FUNCTION_BLOCK PQDXXA_PFN
TITLE =PN Driver
AUTHOR : Parker
VERSION : 1.1


VAR_INPUT
  ENABLE : BOOL ;	//Freigabe des Systems / Enable the System
  ENABLE_P : BOOL ;	//Aktivierung des Druckreglers / Activation of the Pressure Controller
  ENABLE_RAMP : BOOL ;	//Aktivierung des Rampengenerators / Activation of the Ramp Generator
  ENABLE_PL : BOOL ;	//Freigabe der Leistungsbegrenzung über den Feldbus / Enable the Power Limitation
  WQ : REAL ;	//Schwenkwinkelsollwert [%] / Displacement Command Value [%]
  WP : REAL  := 1.000000e+002;	//Drucksollwert [bar] / Pressure Command Value [bar]
  WL : REAL ;	//Leistungssollwert [%] / Horse Power Command [%]
  PAR_CHANGE_IN : STRUCT
   PARVAL : DWORD ;
   PARAMODE : BOOL ;
   ADDRESS : WORD ;
   PARAVALID : BOOL ;
   PARAREAD : BOOL ;
   READULIM : BOOL ;
   READLLIM : BOOL ;
  END_STRUCT ;
  ADR_IN : INT ;	//Eingangsadresse des Slaves / Input adress of the slave
  ADR_OUT : INT ;	//Ausgangsadresse des Slaves / Output adress of the slave
END_VAR
VAR_OUTPUT
  BUS_VALID : BOOL ;	//Buskopplung liefert gültige Werte / Bus Connection Delivers Valid Information
  BUS_ERROR_CODE : BYTE ;	//Fehlercode zur Diagnose / Error Code for Diagnosis
  ERROR : BOOL ;	//Sammelfehler / Common Error Bit
  P_ACTIVE : BOOL ;	//Druckregler aktiv / Pressure Controller Active
  POWER_LIM : BOOL ;	//Leistungsbegrenzung Aktiv / Horse Power Limitation is Active
  READY : BOOL ;	//Allgemeine Betriebsbereitschaft / Operational Readiness
  IQA_ERROR : BOOL ;	//Fehler Magnet A / Error Solenoid A
  IQB_ERROR : BOOL ;	//Fehler Magnet B / Error Solenoid B
  IP_ERROR : BOOL ;	//Fehler Druckventil / Error Pressure Valve
  XQ_ERROR : BOOL ;	//Fehler Schwenkwinkelsensor / Error Displacement Transducer
  XP_ERROR : BOOL ;	//Fehler Drucksensor / Error Pressure Transducer
  HW_ENABLE : BOOL ;	//Enable Eingang des Moduls an PIN8 / Enable Input of the Module at PIN8
  WQFB : REAL ;	//Schwenkwinkelsollwert [%] Rückmeldung / Displacement Command Value [%] Feedback
  XQ : REAL ;	//Schwenkwinkelistwert [%] / Displacement Actual Value [%]
  EQ : REAL ;	//Regelabweichung Schwenkwinkel [%] / Control Error Displacement [%]
  UQ : REAL ;	//Stellsignal Q Ventil [%] / Control Signal Q Valve [%]
  WPFB : REAL ;	//Drucksollwert [bar] Rückmeldung / Pressure Command Value [%] Feedback
  XP : REAL ;	//Druckistwert [bar] / Pressure Actual Value [bar]
  EP : REAL ;	//Regelabweichung Druck [bar] / Control Error Pressure [bar]
  UP : REAL ;	//Stellsignal P Ventil [%] / Control Signal P Valve [%]
  XL : REAL ;	//Schwenkwinkelgrenze durch Leistung [%] / Displacement Limit by Power [%]
  XQ_R : REAL ;	//Schwenkwinkelsensorsignal [V] / Displacement Sensor Signal [V]
  IQ : REAL ;	//Magnetstrom Schwenkwinkelventil [mA] / Solenoid Current Displacement Valve [mA]
  IP : REAL ;	//Magnetstrom Druckventil [mA] / Solenoid Current Pressure Valve [mA]
  PAR_CHANGE_OUT : STRUCT
   PARA_READY : BOOL ;
   BUS_VALID : BOOL ;
   ENABLE : BOOL ;	//Enable Signal for the Controller
   PARA_ACTIVE : BOOL ;
   PARVAL : DWORD ;	//Read out Value
  END_STRUCT ;
END_VAR
VAR
  DATA_IN : ARRAY  [0 .. 31 ] OF BYTE ;
  DATA_OUT : ARRAY  [0 .. 31 ] OF BYTE ;
  LIVEBIT : BOOL ;
  ERROR_TIMER_ON : INT ;
  ERROR_TIMER_OFF : INT ;
END_VAR
VAR_TEMP
  RET_VAL_TMP : INT ;
  TMP_VAL : DWORD ;
  TMP_VAL_WORD : WORD ;
  TMP_BYTE : BYTE ;
  TMP_VAL_REAL : REAL ;
  RCV_ERROR : BOOL ;
  SND_ERROR : BOOL ;
  LIVEBIT_ERROR : BOOL ;
  BUFFERR0V : BOOL ;
  CHKERROR : BOOL ;
  DERROR : BOOL ;
  LIVEBIT_FB : BOOL ;
  i : INT ;
  ADRE : WORD ;
END_VAR
BEGIN
NETWORK
TITLE =

      SET   ;
      SAVE  ;
      =     L     20.1;
      L     #ADR_IN;
      T     #ADRE;
      SAVE  ;

      CALL SFC   14 (
           LADDR                    := #ADRE,
           RET_VAL                  := #RET_VAL_TMP,
           RECORD                   := #DATA_IN);

      L     #RET_VAL_TMP;
      L     0;
      <>I   ;
      =     #RCV_ERROR;
      L     #DATA_IN[0];
      T     #TMP_BYTE;
      U     L      8.0;
      NOT   ;
      =     #DERROR;
      U     L      8.1;
      NOT   ;
      =     #CHKERROR;
      U     L      8.2;
      NOT   ;
      =     #BUFFERR0V;
      U     L      8.3;
      =     #HW_ENABLE;
      U     L      8.4;
      NOT   ;
      =     #ERROR;
      U     L      8.5;
      =     #P_ACTIVE;
      U     L      8.6;
      =     #POWER_LIM;
      U     L      8.7;
      =     #READY;
      U     #ENABLE;
      =     #PAR_CHANGE_OUT.ENABLE;
      L     #DATA_IN[1];
      T     #TMP_BYTE;
      U     L      8.0;
      =     #LIVEBIT_FB;
      U     L      8.1;
      NOT   ;
      =     #IQA_ERROR;
      U     L      8.2;
      NOT   ;
      =     #IQB_ERROR;
      U     L      8.3;
      NOT   ;
      =     #IP_ERROR;
      U     L      8.4;
      NOT   ;
      =     #XQ_ERROR;
      U     L      8.5;
      NOT   ;
      =     #XP_ERROR;
      U     L      8.6;
      =     #PAR_CHANGE_OUT.PARA_READY;
      U     L      8.7;
      =     #PAR_CHANGE_OUT.PARA_ACTIVE;
      U     #LIVEBIT;
      X     #LIVEBIT_FB;
      SPBN  A7d0;
      L     #ERROR_TIMER_ON;
      L     1;
      +I    ;
      SPO   I007;
      SPA   I008;
I007: CLR   ;
      =     L     20.1;
I008: T     #ERROR_TIMER_ON;
      SPA   A7d1;
A7d0: CLR   ;
      U     #LIVEBIT;
      NOT   ;
      =     #LIVEBIT;
      L     0;
      T     #ERROR_TIMER_ON;
A7d1: L     #ERROR_TIMER_ON;
      L     10;
      >=I   ;
      SPBN  A7d2;
      U     #LIVEBIT;
      NOT   ;
      =     #LIVEBIT;
      L     0;
      T     #ERROR_TIMER_ON;
      L     25;
      T     #ERROR_TIMER_OFF;
A7d2: L     #ERROR_TIMER_OFF;
      L     0;
      >I    ;
      SPBN  A7d3;
      L     #ERROR_TIMER_OFF;
      L     1;
      -I    ;
      SPO   I009;
      SPA   I00a;
I009: CLR   ;
      =     L     20.1;
I00a: T     #ERROR_TIMER_OFF;
      SET   ;
      =     #LIVEBIT_ERROR;
      SPA   A7d4;
A7d3: CLR   ;
      =     #LIVEBIT_ERROR;
A7d4: L     0;
      T     #i;
A7d5: L     #i;
      L     1;
      <=I   ;
      SPBN  A7d6;
      L     #i;
      +I    ;
      SPO   I00b;
      SPA   I00c;
I00b: CLR   ;
      =     L     20.1;
I00c: ITD   ;
      L     L#1;
      >=D   ;
      U     L     20.1;
      =     L     20.1;
      TAK   ;
      L     L#2;
      <=D   ;
      U     L     20.1;
      =     L     20.1;
      TAK   ;
      L     L#1;
      -D    ;
      SPO   I00d;
      SPA   I00e;
I00d: CLR   ;
      =     L     20.1;
I00e: L     L#8;
      *D    ;
      SPO   I00f;
      SPA   I010;
I00f: CLR   ;
      =     L     20.1;
I010: L     4;
      TAK   ;
      T     LD    22;
      TAK   ;
      L     #i;
      +I    ;
      SPO   I011;
      SPA   I012;
I011: CLR   ;
      =     L     20.1;
I012: ITD   ;
      L     L#0;
      >=D   ;
      U     L     20.1;
      =     L     20.1;
      TAK   ;
      L     L#31;
      <=D   ;
      U     L     20.1;
      =     L     20.1;
      TAK   ;
      L     L#8;
      *D    ;
      SPO   I013;
      SPA   I014;
I013: CLR   ;
      =     L     20.1;
I014: TAR2  ;
      +D    ;
      SPO   I015;
      SPA   I016;
I015: CLR   ;
      =     L     20.1;
I016: LAR1  ;
      L     DIB [AR1,P#86.0];
      LAR1  LD    22;
      T     LB [AR1,P#6.0];
      L     #i;
      L     1;
      +I    ;
      SPO   I017;
      SPA   I018;
I017: CLR   ;
      =     L     20.1;
I018: T     #i;
      SPA   A7d5;
A7d6: L     #TMP_VAL_WORD;
      CLR   ;
      U     L     20.1;
      SAVE  ;
      ITD   ;
      DTR   ;
      T     #TMP_VAL_REAL;
      SAVE  ;
      L     1.638300e+002;
      /R    ;
      SPO   I019;
      SPA   I01a;
I019: CLR   ;
      =     L     20.1;
I01a: T     #WQFB;
      L     0;
      T     #i;
A7d7: L     #i;
      L     1;
      <=I   ;
      SPBN  A7d8;
      L     #i;
      +I    ;
      SPO   I01b;
      SPA   I01c;
I01b: CLR   ;
      =     L     20.1;
I01c: ITD   ;
      L     L#1;
      >=D   ;
      U     L     20.1;
      =     L     20.1;
      TAK   ;
      L     L#2;
      <=D   ;
      U     L     20.1;
      =     L     20.1;
      TAK   ;
      L     L#1;
      -D    ;
      SPO   I01d;
      SPA   I01e;
I01d: CLR   ;
      =     L     20.1;
I01e: L     L#8;
      *D    ;
      SPO   I01f;
      SPA   I020;
I01f: CLR   ;
      =     L     20.1;
I020: L     6;
      TAK   ;
      T     LD    22;
      TAK   ;
      L     #i;
      +I    ;
      SPO   I021;
      SPA   I022;
I021: CLR   ;
      =     L     20.1;
I022: ITD   ;
      L     L#0;
      >=D   ;
      U     L     20.1;
      =     L     20.1;
      TAK   ;
      L     L#31;
      <=D   ;
      U     L     20.1;
      =     L     20.1;
      TAK   ;
      L     L#8;
      *D    ;
      SPO   I023;
      SPA   I024;
I023: CLR   ;
      =     L     20.1;
I024: TAR2  ;
      +D    ;
      SPO   I025;
      SPA   I026;
I025: CLR   ;
      =     L     20.1;
I026: LAR1  ;
      L     DIB [AR1,P#86.0];
      LAR1  LD    22;
      T     LB [AR1,P#6.0];
      L     #i;
      L     1;
      +I    ;
      SPO   I027;
      SPA   I028;
I027: CLR   ;
      =     L     20.1;
I028: T     #i;
      SPA   A7d7;
A7d8: L     #TMP_VAL_WORD;
      CLR   ;
      U     L     20.1;
      SAVE  ;
      ITD   ;
      DTR   ;
      T     #TMP_VAL_REAL;
      SAVE  ;
      L     1.638300e+002;
      /R    ;
      SPO   I029;
      SPA   I02a;
I029: CLR   ;
      =     L     20.1;
I02a: T     #XQ;
      L     0;
      T     #i;
A7d9: L     #i;
      L     1;
      <=I   ;
      SPBN  A7da;
      L     #i;
      +I    ;
      SPO   I02b;
      SPA   I02c;
I02b: CLR   ;
      =     L     20.1;
I02c: ITD   ;
      L     L#1;
      >=D   ;
      U     L     20.1;
      =     L     20.1;
      TAK   ;
      L     L#2;
      <=D   ;
      U     L     20.1;
      =     L     20.1;
      TAK   ;
      L     L#1;
      -D    ;
      SPO   I02d;
      SPA   I02e;
I02d: CLR   ;
      =     L     20.1;
I02e: L     L#8;
      *D    ;
      SPO   I02f;
      SPA   I030;
I02f: CLR   ;
      =     L     20.1;
I030: L     8;
      TAK   ;
      T     LD    22;
      TAK   ;
      L     #i;
      +I    ;
      SPO   I031;
      SPA   I032;
I031: CLR   ;
      =     L     20.1;
I032: ITD   ;
      L     L#0;
      >=D   ;
      U     L     20.1;
      =     L     20.1;
      TAK   ;
      L     L#31;
      <=D   ;
      U     L     20.1;
      =     L     20.1;
      TAK   ;
      L     L#8;
      *D    ;
      SPO   I033;
      SPA   I034;
I033: CLR   ;
      =     L     20.1;
I034: TAR2  ;
      +D    ;
      SPO   I035;
      SPA   I036;
I035: CLR   ;
      =     L     20.1;
I036: LAR1  ;
      L     DIB [AR1,P#86.0];
      LAR1  LD    22;
      T     LB [AR1,P#6.0];
      L     #i;
      L     1;
      +I    ;
      SPO   I037;
      SPA   I038;
I037: CLR   ;
      =     L     20.1;
I038: T     #i;
      SPA   A7d9;
A7da: L     #TMP_VAL_WORD;
      CLR   ;
      U     L     20.1;
      SAVE  ;
      ITD   ;
      DTR   ;
      T     #TMP_VAL_REAL;
      SAVE  ;
      L     1.638300e+002;
      /R    ;
      SPO   I039;
      SPA   I03a;
I039: CLR   ;
      =     L     20.1;
I03a: T     #EQ;
      L     0;
      T     #i;
A7db: L     #i;
      L     1;
      <=I   ;
      SPBN  A7dc;
      L     #i;
      +I    ;
      SPO   I03b;
      SPA   I03c;
I03b: CLR   ;
      =     L     20.1;
I03c: ITD   ;
      L     L#1;
      >=D   ;
      U     L     20.1;
      =     L     20.1;
      TAK   ;
      L     L#2;
      <=D   ;
      U     L     20.1;
      =     L     20.1;
      TAK   ;
      L     L#1;
      -D    ;
      SPO   I03d;
      SPA   I03e;
I03d: CLR   ;
      =     L     20.1;
I03e: L     L#8;
      *D    ;
      SPO   I03f;
      SPA   I040;
I03f: CLR   ;
      =     L     20.1;
I040: L     10;
      TAK   ;
      T     LD    22;
      TAK   ;
      L     #i;
      +I    ;
      SPO   I041;
      SPA   I042;
I041: CLR   ;
      =     L     20.1;
I042: ITD   ;
      L     L#0;
      >=D   ;
      U     L     20.1;
      =     L     20.1;
      TAK   ;
      L     L#31;
      <=D   ;
      U     L     20.1;
      =     L     20.1;
      TAK   ;
      L     L#8;
      *D    ;
      SPO   I043;
      SPA   I044;
I043: CLR   ;
      =     L     20.1;
I044: TAR2  ;
      +D    ;
      SPO   I045;
      SPA   I046;
I045: CLR   ;
      =     L     20.1;
I046: LAR1  ;
      L     DIB [AR1,P#86.0];
      LAR1  LD    22;
      T     LB [AR1,P#6.0];
      L     #i;
      L     1;
      +I    ;
      SPO   I047;
      SPA   I048;
I047: CLR   ;
      =     L     20.1;
I048: T     #i;
      SPA   A7db;
A7dc: L     #TMP_VAL_WORD;
      CLR   ;
      U     L     20.1;
      SAVE  ;
      ITD   ;
      DTR   ;
      T     #TMP_VAL_REAL;
      SAVE  ;
      L     1.638300e+002;
      /R    ;
      SPO   I049;
      SPA   I04a;
I049: CLR   ;
      =     L     20.1;
I04a: T     #UQ;
      L     0;
      T     #i;
A7dd: L     #i;
      L     1;
      <=I   ;
      SPBN  A7de;
      L     #i;
      +I    ;
      SPO   I04b;
      SPA   I04c;
I04b: CLR   ;
      =     L     20.1;
I04c: ITD   ;
      L     L#1;
      >=D   ;
      U     L     20.1;
      =     L     20.1;
      TAK   ;
      L     L#2;
      <=D   ;
      U     L     20.1;
      =     L     20.1;
      TAK   ;
      L     L#1;
      -D    ;
      SPO   I04d;
      SPA   I04e;
I04d: CLR   ;
      =     L     20.1;
I04e: L     L#8;
      *D    ;
      SPO   I04f;
      SPA   I050;
I04f: CLR   ;
      =     L     20.1;
I050: L     12;
      TAK   ;
      T     LD    22;
      TAK   ;
      L     #i;
      +I    ;
      SPO   I051;
      SPA   I052;
I051: CLR   ;
      =     L     20.1;
I052: ITD   ;
      L     L#0;
      >=D   ;
      U     L     20.1;
      =     L     20.1;
      TAK   ;
      L     L#31;
      <=D   ;
      U     L     20.1;
      =     L     20.1;
      TAK   ;
      L     L#8;
      *D    ;
      SPO   I053;
      SPA   I054;
I053: CLR   ;
      =     L     20.1;
I054: TAR2  ;
      +D    ;
      SPO   I055;
      SPA   I056;
I055: CLR   ;
      =     L     20.1;
I056: LAR1  ;
      L     DIB [AR1,P#86.0];
      LAR1  LD    22;
      T     LB [AR1,P#6.0];
      L     #i;
      L     1;
      +I    ;
      SPO   I057;
      SPA   I058;
I057: CLR   ;
      =     L     20.1;
I058: T     #i;
      SPA   A7dd;
A7de: L     #TMP_VAL_WORD;
      CLR   ;
      U     L     20.1;
      SAVE  ;
      ITD   ;
      DTR   ;
      T     #TMP_VAL_REAL;
      SAVE  ;
      L     1.000000e+001;
      /R    ;
      SPO   I059;
      SPA   I05a;
I059: CLR   ;
      =     L     20.1;
I05a: T     #WPFB;
      L     0;
      T     #i;
A7df: L     #i;
      L     1;
      <=I   ;
      SPBN  A7e0;
      L     #i;
      +I    ;
      SPO   I05b;
      SPA   I05c;
I05b: CLR   ;
      =     L     20.1;
I05c: ITD   ;
      L     L#1;
      >=D   ;
      U     L     20.1;
      =     L     20.1;
      TAK   ;
      L     L#2;
      <=D   ;
      U     L     20.1;
      =     L     20.1;
      TAK   ;
      L     L#1;
      -D    ;
      SPO   I05d;
      SPA   I05e;
I05d: CLR   ;
      =     L     20.1;
I05e: L     L#8;
      *D    ;
      SPO   I05f;
      SPA   I060;
I05f: CLR   ;
      =     L     20.1;
I060: L     14;
      TAK   ;
      T     LD    22;
      TAK   ;
      L     #i;
      +I    ;
      SPO   I061;
      SPA   I062;
I061: CLR   ;
      =     L     20.1;
I062: ITD   ;
      L     L#0;
      >=D   ;
      U     L     20.1;
      =     L     20.1;
      TAK   ;
      L     L#31;
      <=D   ;
      U     L     20.1;
      =     L     20.1;
      TAK   ;
      L     L#8;
      *D    ;
      SPO   I063;
      SPA   I064;
I063: CLR   ;
      =     L     20.1;
I064: TAR2  ;
      +D    ;
      SPO   I065;
      SPA   I066;
I065: CLR   ;
      =     L     20.1;
I066: LAR1  ;
      L     DIB [AR1,P#86.0];
      LAR1  LD    22;
      T     LB [AR1,P#6.0];
      L     #i;
      L     1;
      +I    ;
      SPO   I067;
      SPA   I068;
I067: CLR   ;
      =     L     20.1;
I068: T     #i;
      SPA   A7df;
A7e0: L     #TMP_VAL_WORD;
      CLR   ;
      U     L     20.1;
      SAVE  ;
      ITD   ;
      DTR   ;
      T     #TMP_VAL_REAL;
      SAVE  ;
      L     1.000000e+001;
      /R    ;
      SPO   I069;
      SPA   I06a;
I069: CLR   ;
      =     L     20.1;
I06a: T     #XP;
      L     0;
      T     #i;
A7e1: L     #i;
      L     1;
      <=I   ;
      SPBN  A7e2;
      L     #i;
      +I    ;
      SPO   I06b;
      SPA   I06c;
I06b: CLR   ;
      =     L     20.1;
I06c: ITD   ;
      L     L#1;
      >=D   ;
      U     L     20.1;
      =     L     20.1;
      TAK   ;
      L     L#2;
      <=D   ;
      U     L     20.1;
      =     L     20.1;
      TAK   ;
      L     L#1;
      -D    ;
      SPO   I06d;
      SPA   I06e;
I06d: CLR   ;
      =     L     20.1;
I06e: L     L#8;
      *D    ;
      SPO   I06f;
      SPA   I070;
I06f: CLR   ;
      =     L     20.1;
I070: L     16;
      TAK   ;
      T     LD    22;
      TAK   ;
      L     #i;
      +I    ;
      SPO   I071;
      SPA   I072;
I071: CLR   ;
      =     L     20.1;
I072: ITD   ;
      L     L#0;
      >=D   ;
      U     L     20.1;
      =     L     20.1;
      TAK   ;
      L     L#31;
      <=D   ;
      U     L     20.1;
      =     L     20.1;
      TAK   ;
      L     L#8;
      *D    ;
      SPO   I073;
      SPA   I074;
I073: CLR   ;
      =     L     20.1;
I074: TAR2  ;
      +D    ;
      SPO   I075;
      SPA   I076;
I075: CLR   ;
      =     L     20.1;
I076: LAR1  ;
      L     DIB [AR1,P#86.0];
      LAR1  LD    22;
      T     LB [AR1,P#6.0];
      L     #i;
      L     1;
      +I    ;
      SPO   I077;
      SPA   I078;
I077: CLR   ;
      =     L     20.1;
I078: T     #i;
      SPA   A7e1;
A7e2: L     #TMP_VAL_WORD;
      CLR   ;
      U     L     20.1;
      SAVE  ;
      ITD   ;
      DTR   ;
      T     #TMP_VAL_REAL;
      SAVE  ;
      L     1.000000e+001;
      /R    ;
      SPO   I079;
      SPA   I07a;
I079: CLR   ;
      =     L     20.1;
I07a: T     #EP;
      L     0;
      T     #i;
A7e3: L     #i;
      L     1;
      <=I   ;
      SPBN  A7e4;
      L     #i;
      +I    ;
      SPO   I07b;
      SPA   I07c;
I07b: CLR   ;
      =     L     20.1;
I07c: ITD   ;
      L     L#1;
      >=D   ;
      U     L     20.1;
      =     L     20.1;
      TAK   ;
      L     L#2;
      <=D   ;
      U     L     20.1;
      =     L     20.1;
      TAK   ;
      L     L#1;
      -D    ;
      SPO   I07d;
      SPA   I07e;
I07d: CLR   ;
      =     L     20.1;
I07e: L     L#8;
      *D    ;
      SPO   I07f;
      SPA   I080;
I07f: CLR   ;
      =     L     20.1;
I080: L     18;
      TAK   ;
      T     LD    22;
      TAK   ;
      L     #i;
      +I    ;
      SPO   I081;
      SPA   I082;
I081: CLR   ;
      =     L     20.1;
I082: ITD   ;
      L     L#0;
      >=D   ;
      U     L     20.1;
      =     L     20.1;
      TAK   ;
      L     L#31;
      <=D   ;
      U     L     20.1;
      =     L     20.1;
      TAK   ;
      L     L#8;
      *D    ;
      SPO   I083;
      SPA   I084;
I083: CLR   ;
      =     L     20.1;
I084: TAR2  ;
      +D    ;
      SPO   I085;
      SPA   I086;
I085: CLR   ;
      =     L     20.1;
I086: LAR1  ;
      L     DIB [AR1,P#86.0];
      LAR1  LD    22;
      T     LB [AR1,P#6.0];
      L     #i;
      L     1;
      +I    ;
      SPO   I087;
      SPA   I088;
I087: CLR   ;
      =     L     20.1;
I088: T     #i;
      SPA   A7e3;
A7e4: L     #TMP_VAL_WORD;
      CLR   ;
      U     L     20.1;
      SAVE  ;
      ITD   ;
      DTR   ;
      T     #TMP_VAL_REAL;
      SAVE  ;
      L     1.638300e+002;
      /R    ;
      SPO   I089;
      SPA   I08a;
I089: CLR   ;
      =     L     20.1;
I08a: T     #UP;
      L     0;
      T     #i;
A7e5: L     #i;
      L     1;
      <=I   ;
      SPBN  A7e6;
      L     #i;
      +I    ;
      SPO   I08b;
      SPA   I08c;
I08b: CLR   ;
      =     L     20.1;
I08c: ITD   ;
      L     L#1;
      >=D   ;
      U     L     20.1;
      =     L     20.1;
      TAK   ;
      L     L#2;
      <=D   ;
      U     L     20.1;
      =     L     20.1;
      TAK   ;
      L     L#1;
      -D    ;
      SPO   I08d;
      SPA   I08e;
I08d: CLR   ;
      =     L     20.1;
I08e: L     L#8;
      *D    ;
      SPO   I08f;
      SPA   I090;
I08f: CLR   ;
      =     L     20.1;
I090: L     20;
      TAK   ;
      T     LD    22;
      TAK   ;
      L     #i;
      +I    ;
      SPO   I091;
      SPA   I092;
I091: CLR   ;
      =     L     20.1;
I092: ITD   ;
      L     L#0;
      >=D   ;
      U     L     20.1;
      =     L     20.1;
      TAK   ;
      L     L#31;
      <=D   ;
      U     L     20.1;
      =     L     20.1;
      TAK   ;
      L     L#8;
      *D    ;
      SPO   I093;
      SPA   I094;
I093: CLR   ;
      =     L     20.1;
I094: TAR2  ;
      +D    ;
      SPO   I095;
      SPA   I096;
I095: CLR   ;
      =     L     20.1;
I096: LAR1  ;
      L     DIB [AR1,P#86.0];
      LAR1  LD    22;
      T     LB [AR1,P#6.0];
      L     #i;
      L     1;
      +I    ;
      SPO   I097;
      SPA   I098;
I097: CLR   ;
      =     L     20.1;
I098: T     #i;
      SPA   A7e5;
A7e6: L     #TMP_VAL_WORD;
      CLR   ;
      U     L     20.1;
      SAVE  ;
      ITD   ;
      DTR   ;
      T     #TMP_VAL_REAL;
      SAVE  ;
      L     1.638300e+002;
      /R    ;
      SPO   I099;
      SPA   I09a;
I099: CLR   ;
      =     L     20.1;
I09a: T     #XL;
      L     0;
      T     #i;
A7e7: L     #i;
      L     1;
      <=I   ;
      SPBN  A7e8;
      L     #i;
      +I    ;
      SPO   I09b;
      SPA   I09c;
I09b: CLR   ;
      =     L     20.1;
I09c: ITD   ;
      L     L#1;
      >=D   ;
      U     L     20.1;
      =     L     20.1;
      TAK   ;
      L     L#2;
      <=D   ;
      U     L     20.1;
      =     L     20.1;
      TAK   ;
      L     L#1;
      -D    ;
      SPO   I09d;
      SPA   I09e;
I09d: CLR   ;
      =     L     20.1;
I09e: L     L#8;
      *D    ;
      SPO   I09f;
      SPA   I0a0;
I09f: CLR   ;
      =     L     20.1;
I0a0: L     22;
      TAK   ;
      T     LD    22;
      TAK   ;
      L     #i;
      +I    ;
      SPO   I0a1;
      SPA   I0a2;
I0a1: CLR   ;
      =     L     20.1;
I0a2: ITD   ;
      L     L#0;
      >=D   ;
      U     L     20.1;
      =     L     20.1;
      TAK   ;
      L     L#31;
      <=D   ;
      U     L     20.1;
      =     L     20.1;
      TAK   ;
      L     L#8;
      *D    ;
      SPO   I0a3;
      SPA   I0a4;
I0a3: CLR   ;
      =     L     20.1;
I0a4: TAR2  ;
      +D    ;
      SPO   I0a5;
      SPA   I0a6;
I0a5: CLR   ;
      =     L     20.1;
I0a6: LAR1  ;
      L     DIB [AR1,P#86.0];
      LAR1  LD    22;
      T     LB [AR1,P#6.0];
      L     #i;
      L     1;
      +I    ;
      SPO   I0a7;
      SPA   I0a8;
I0a7: CLR   ;
      =     L     20.1;
I0a8: T     #i;
      SPA   A7e7;
A7e8: L     #TMP_VAL_WORD;
      CLR   ;
      U     L     20.1;
      SAVE  ;
      ITD   ;
      DTR   ;
      T     #TMP_VAL_REAL;
      SAVE  ;
      L     1.000000e-002;
      *R    ;
      SPO   I0a9;
      SPA   I0aa;
I0a9: CLR   ;
      =     L     20.1;
I0aa: T     #XQ_R;
      L     0;
      T     #i;
A7e9: L     #i;
      L     1;
      <=I   ;
      SPBN  A7ea;
      L     #i;
      +I    ;
      SPO   I0ab;
      SPA   I0ac;
I0ab: CLR   ;
      =     L     20.1;
I0ac: ITD   ;
      L     L#1;
      >=D   ;
      U     L     20.1;
      =     L     20.1;
      TAK   ;
      L     L#2;
      <=D   ;
      U     L     20.1;
      =     L     20.1;
      TAK   ;
      L     L#1;
      -D    ;
      SPO   I0ad;
      SPA   I0ae;
I0ad: CLR   ;
      =     L     20.1;
I0ae: L     L#8;
      *D    ;
      SPO   I0af;
      SPA   I0b0;
I0af: CLR   ;
      =     L     20.1;
I0b0: L     24;
      TAK   ;
      T     LD    22;
      TAK   ;
      L     #i;
      +I    ;
      SPO   I0b1;
      SPA   I0b2;
I0b1: CLR   ;
      =     L     20.1;
I0b2: ITD   ;
      L     L#0;
      >=D   ;
      U     L     20.1;
      =     L     20.1;
      TAK   ;
      L     L#31;
      <=D   ;
      U     L     20.1;
      =     L     20.1;
      TAK   ;
      L     L#8;
      *D    ;
      SPO   I0b3;
      SPA   I0b4;
I0b3: CLR   ;
      =     L     20.1;
I0b4: TAR2  ;
      +D    ;
      SPO   I0b5;
      SPA   I0b6;
I0b5: CLR   ;
      =     L     20.1;
I0b6: LAR1  ;
      L     DIB [AR1,P#86.0];
      LAR1  LD    22;
      T     LB [AR1,P#6.0];
      L     #i;
      L     1;
      +I    ;
      SPO   I0b7;
      SPA   I0b8;
I0b7: CLR   ;
      =     L     20.1;
I0b8: T     #i;
      SPA   A7e9;
A7ea: L     #TMP_VAL_WORD;
      CLR   ;
      U     L     20.1;
      SAVE  ;
      ITD   ;
      DTR   ;
      T     #IQ;
      SAVE  ;
      L     0;
      T     #i;
A7eb: L     #i;
      L     1;
      <=I   ;
      SPBN  A7ec;
      L     #i;
      +I    ;
      SPO   I0b9;
      SPA   I0ba;
I0b9: CLR   ;
      =     L     20.1;
I0ba: ITD   ;
      L     L#1;
      >=D   ;
      U     L     20.1;
      =     L     20.1;
      TAK   ;
      L     L#2;
      <=D   ;
      U     L     20.1;
      =     L     20.1;
      TAK   ;
      L     L#1;
      -D    ;
      SPO   I0bb;
      SPA   I0bc;
I0bb: CLR   ;
      =     L     20.1;
I0bc: L     L#8;
      *D    ;
      SPO   I0bd;
      SPA   I0be;
I0bd: CLR   ;
      =     L     20.1;
I0be: L     26;
      TAK   ;
      T     LD    22;
      TAK   ;
      L     #i;
      +I    ;
      SPO   I0bf;
      SPA   I0c0;
I0bf: CLR   ;
      =     L     20.1;
I0c0: ITD   ;
      L     L#0;
      >=D   ;
      U     L     20.1;
      =     L     20.1;
      TAK   ;
      L     L#31;
      <=D   ;
      U     L     20.1;
      =     L     20.1;
      TAK   ;
      L     L#8;
      *D    ;
      SPO   I0c1;
      SPA   I0c2;
I0c1: CLR   ;
      =     L     20.1;
I0c2: TAR2  ;
      +D    ;
      SPO   I0c3;
      SPA   I0c4;
I0c3: CLR   ;
      =     L     20.1;
I0c4: LAR1  ;
      L     DIB [AR1,P#86.0];
      LAR1  LD    22;
      T     LB [AR1,P#6.0];
      L     #i;
      L     1;
      +I    ;
      SPO   I0c5;
      SPA   I0c6;
I0c5: CLR   ;
      =     L     20.1;
I0c6: T     #i;
      SPA   A7eb;
A7ec: L     #TMP_VAL_WORD;
      CLR   ;
      U     L     20.1;
      SAVE  ;
      ITD   ;
      DTR   ;
      T     #IP;
      SAVE  ;
      L     0;
      T     #i;
A7ed: L     #i;
      L     3;
      <=I   ;
      SPBN  A7ee;
      L     1;
      L     #i;
      +I    ;
      SPO   I0c7;
      SPA   I0c8;
I0c7: CLR   ;
      =     L     20.1;
I0c8: ITD   ;
      L     L#1;
      >=D   ;
      U     L     20.1;
      =     L     20.1;
      TAK   ;
      L     L#4;
      <=D   ;
      U     L     20.1;
      =     L     20.1;
      TAK   ;
      L     L#1;
      -D    ;
      SPO   I0c9;
      SPA   I0ca;
I0c9: CLR   ;
      =     L     20.1;
I0ca: L     L#8;
      *D    ;
      SPO   I0cb;
      SPA   I0cc;
I0cb: CLR   ;
      =     L     20.1;
I0cc: L     28;
      TAK   ;
      T     LD    22;
      TAK   ;
      L     #i;
      +I    ;
      SPO   I0cd;
      SPA   I0ce;
I0cd: CLR   ;
      =     L     20.1;
I0ce: ITD   ;
      L     L#0;
      >=D   ;
      U     L     20.1;
      =     L     20.1;
      TAK   ;
      L     L#31;
      <=D   ;
      U     L     20.1;
      =     L     20.1;
      TAK   ;
      L     L#8;
      *D    ;
      SPO   I0cf;
      SPA   I0d0;
I0cf: CLR   ;
      =     L     20.1;
I0d0: TAR2  ;
      +D    ;
      SPO   I0d1;
      SPA   I0d2;
I0d1: CLR   ;
      =     L     20.1;
I0d2: LAR1  ;
      L     DIB [AR1,P#86.0];
      LAR1  LD    22;
      T     LB [AR1,P#2.0];
      L     #i;
      L     1;
      +I    ;
      SPO   I0d3;
      SPA   I0d4;
I0d3: CLR   ;
      =     L     20.1;
I0d4: T     #i;
      SPA   A7ed;
A7ee: L     #TMP_VAL;
      T     #PAR_CHANGE_OUT.PARVAL;
      CLR   ;
      =     L      8.0;
      =     L      8.1;
      =     L      8.2;
      =     L      8.3;
      U     #ENABLE_PL;
      =     L      8.4;
      U     #ENABLE_RAMP;
      =     L      8.5;
      U     #ENABLE_P;
      =     L      8.6;
      U     #ENABLE;
      =     L      8.7;
      L     #TMP_BYTE;
      T     #DATA_OUT[0];
      U     #LIVEBIT;
      =     L      8.0;
      CLR   ;
      =     L      8.1;
      =     L      8.2;
      U     #PAR_CHANGE_IN.READLLIM;
      =     L      8.3;
      U     #PAR_CHANGE_IN.READULIM;
      =     L      8.4;
      U     #PAR_CHANGE_IN.PARAREAD;
      =     L      8.5;
      U     #PAR_CHANGE_IN.PARAVALID;
      =     L      8.6;
      U     #PAR_CHANGE_IN.PARAMODE;
      =     L      8.7;
      L     #TMP_BYTE;
      T     #DATA_OUT[1];
      L     #WQ;
      T     #TMP_VAL_REAL;
      L     0.000000e+000;
      <R    ;
      SPBN  A7ef;
      T     #TMP_VAL_REAL;
      SPA   A7f1;
A7ef: L     #TMP_VAL_REAL;
      L     1.000000e+002;
      >R    ;
      SPBN  A7f1;
      T     #TMP_VAL_REAL;
A7f1: L     #TMP_VAL_REAL;
      L     1.638300e+002;
      *R    ;
      SPO   I0d5;
      SPA   I0d6;
I0d5: CLR   ;
      =     L     20.1;
I0d6: T     #TMP_VAL_REAL;
      RND   ;
      SPO   I0d7;
      SPA   I0d8;
I0d7: CLR   ;
      =     L     20.1;
I0d8: CLR   ;
      U     L     20.1;
      SAVE  ;
      T     #TMP_VAL;
      SAVE  ;
      L     0;
      T     #i;
A7f2: L     #i;
      L     1;
      <=I   ;
      SPBN  A7f3;
      L     4;
      L     #i;
      +I    ;
      SPO   I0d9;
      SPA   I0da;
I0d9: CLR   ;
      =     L     20.1;
I0da: ITD   ;
      L     L#0;
      >=D   ;
      U     L     20.1;
      =     L     20.1;
      TAK   ;
      L     L#31;
      <=D   ;
      U     L     20.1;
      =     L     20.1;
      TAK   ;
      L     L#8;
      *D    ;
      SPO   I0db;
      SPA   I0dc;
I0db: CLR   ;
      =     L     20.1;
I0dc: TAR2  ;
      +D    ;
      SPO   I0dd;
      SPA   I0de;
I0dd: CLR   ;
      =     L     20.1;
I0de: L     3;
      TAK   ;
      T     LD    22;
      TAK   ;
      L     #i;
      +I    ;
      SPO   I0df;
      SPA   I0e0;
I0df: CLR   ;
      =     L     20.1;
I0e0: ITD   ;
      L     L#1;
      >=D   ;
      U     L     20.1;
      =     L     20.1;
      TAK   ;
      L     L#4;
      <=D   ;
      U     L     20.1;
      =     L     20.1;
      TAK   ;
      L     L#1;
      -D    ;
      SPO   I0e1;
      SPA   I0e2;
I0e1: CLR   ;
      =     L     20.1;
I0e2: L     L#8;
      *D    ;
      SPO   I0e3;
      SPA   I0e4;
I0e3: CLR   ;
      =     L     20.1;
I0e4: LAR1  ;
      L     LB [AR1,P#2.0];
      LAR1  LD    22;
      T     DIB [AR1,P#118.0];
      L     #i;
      L     1;
      +I    ;
      SPO   I0e5;
      SPA   I0e6;
I0e5: CLR   ;
      =     L     20.1;
I0e6: T     #i;
      SPA   A7f2;
A7f3: L     #WP;
      T     #TMP_VAL_REAL;
      L     0.000000e+000;
      <R    ;
      SPBN  A7f4;
      T     #TMP_VAL_REAL;
      SPA   A7f6;
A7f4: L     #TMP_VAL_REAL;
      L     1.000000e+003;
      >R    ;
      SPBN  A7f6;
      T     #TMP_VAL_REAL;
A7f6: L     #TMP_VAL_REAL;
      L     1.000000e+001;
      *R    ;
      SPO   I0e7;
      SPA   I0e8;
I0e7: CLR   ;
      =     L     20.1;
I0e8: T     #TMP_VAL_REAL;
      RND   ;
      SPO   I0e9;
      SPA   I0ea;
I0e9: CLR   ;
      =     L     20.1;
I0ea: CLR   ;
      U     L     20.1;
      SAVE  ;
      T     #TMP_VAL;
      SAVE  ;
      L     0;
      T     #i;
A7f7: L     #i;
      L     1;
      <=I   ;
      SPBN  A7f8;
      L     6;
      L     #i;
      +I    ;
      SPO   I0eb;
      SPA   I0ec;
I0eb: CLR   ;
      =     L     20.1;
I0ec: ITD   ;
      L     L#0;
      >=D   ;
      U     L     20.1;
      =     L     20.1;
      TAK   ;
      L     L#31;
      <=D   ;
      U     L     20.1;
      =     L     20.1;
      TAK   ;
      L     L#8;
      *D    ;
      SPO   I0ed;
      SPA   I0ee;
I0ed: CLR   ;
      =     L     20.1;
I0ee: TAR2  ;
      +D    ;
      SPO   I0ef;
      SPA   I0f0;
I0ef: CLR   ;
      =     L     20.1;
I0f0: L     3;
      TAK   ;
      T     LD    22;
      TAK   ;
      L     #i;
      +I    ;
      SPO   I0f1;
      SPA   I0f2;
I0f1: CLR   ;
      =     L     20.1;
I0f2: ITD   ;
      L     L#1;
      >=D   ;
      U     L     20.1;
      =     L     20.1;
      TAK   ;
      L     L#4;
      <=D   ;
      U     L     20.1;
      =     L     20.1;
      TAK   ;
      L     L#1;
      -D    ;
      SPO   I0f3;
      SPA   I0f4;
I0f3: CLR   ;
      =     L     20.1;
I0f4: L     L#8;
      *D    ;
      SPO   I0f5;
      SPA   I0f6;
I0f5: CLR   ;
      =     L     20.1;
I0f6: LAR1  ;
      L     LB [AR1,P#2.0];
      LAR1  LD    22;
      T     DIB [AR1,P#118.0];
      L     #i;
      L     1;
      +I    ;
      SPO   I0f7;
      SPA   I0f8;
I0f7: CLR   ;
      =     L     20.1;
I0f8: T     #i;
      SPA   A7f7;
A7f8: L     #WL;
      T     #TMP_VAL_REAL;
      L     0.000000e+000;
      <R    ;
      SPBN  A7f9;
      T     #TMP_VAL_REAL;
      SPA   A7fb;
A7f9: L     #TMP_VAL_REAL;
      L     1.000000e+002;
      >R    ;
      SPBN  A7fb;
      T     #TMP_VAL_REAL;
A7fb: L     #TMP_VAL_REAL;
      L     1.638300e+002;
      *R    ;
      SPO   I0f9;
      SPA   I0fa;
I0f9: CLR   ;
      =     L     20.1;
I0fa: T     #TMP_VAL_REAL;
      RND   ;
      SPO   I0fb;
      SPA   I0fc;
I0fb: CLR   ;
      =     L     20.1;
I0fc: CLR   ;
      U     L     20.1;
      SAVE  ;
      T     #TMP_VAL;
      SAVE  ;
      L     0;
      T     #i;
A7fc: L     #i;
      L     1;
      <=I   ;
      SPBN  A7fd;
      L     8;
      L     #i;
      +I    ;
      SPO   I0fd;
      SPA   I0fe;
I0fd: CLR   ;
      =     L     20.1;
I0fe: ITD   ;
      L     L#0;
      >=D   ;
      U     L     20.1;
      =     L     20.1;
      TAK   ;
      L     L#31;
      <=D   ;
      U     L     20.1;
      =     L     20.1;
      TAK   ;
      L     L#8;
      *D    ;
      SPO   I0ff;
      SPA   I100;
I0ff: CLR   ;
      =     L     20.1;
I100: TAR2  ;
      +D    ;
      SPO   I101;
      SPA   I102;
I101: CLR   ;
      =     L     20.1;
I102: L     3;
      TAK   ;
      T     LD    22;
      TAK   ;
      L     #i;
      +I    ;
      SPO   I103;
      SPA   I104;
I103: CLR   ;
      =     L     20.1;
I104: ITD   ;
      L     L#1;
      >=D   ;
      U     L     20.1;
      =     L     20.1;
      TAK   ;
      L     L#4;
      <=D   ;
      U     L     20.1;
      =     L     20.1;
      TAK   ;
      L     L#1;
      -D    ;
      SPO   I105;
      SPA   I106;
I105: CLR   ;
      =     L     20.1;
I106: L     L#8;
      *D    ;
      SPO   I107;
      SPA   I108;
I107: CLR   ;
      =     L     20.1;
I108: LAR1  ;
      L     LB [AR1,P#2.0];
      LAR1  LD    22;
      T     DIB [AR1,P#118.0];
      L     #i;
      L     1;
      +I    ;
      SPO   I109;
      SPA   I10a;
I109: CLR   ;
      =     L     20.1;
I10a: T     #i;
      SPA   A7fc;
A7fd: L     #PAR_CHANGE_IN.ADDRESS;
      UD    DW#16#FFFF;
      T     #TMP_VAL;
      CLR   ;
      U     L     20.1;
      SAVE  ;
      L     0;
      T     #i;
A7fe: L     #i;
      L     1;
      <=I   ;
      SPBN  A7ff;
      L     30;
      L     #i;
      +I    ;
      SPO   I10b;
      SPA   I10c;
I10b: CLR   ;
      =     L     20.1;
I10c: ITD   ;
      L     L#0;
      >=D   ;
      U     L     20.1;
      =     L     20.1;
      TAK   ;
      L     L#31;
      <=D   ;
      U     L     20.1;
      =     L     20.1;
      TAK   ;
      L     L#8;
      *D    ;
      SPO   I10d;
      SPA   I10e;
I10d: CLR   ;
      =     L     20.1;
I10e: TAR2  ;
      +D    ;
      SPO   I10f;
      SPA   I110;
I10f: CLR   ;
      =     L     20.1;
I110: L     3;
      TAK   ;
      T     LD    22;
      TAK   ;
      L     #i;
      +I    ;
      SPO   I111;
      SPA   I112;
I111: CLR   ;
      =     L     20.1;
I112: ITD   ;
      L     L#1;
      >=D   ;
      U     L     20.1;
      =     L     20.1;
      TAK   ;
      L     L#4;
      <=D   ;
      U     L     20.1;
      =     L     20.1;
      TAK   ;
      L     L#1;
      -D    ;
      SPO   I113;
      SPA   I114;
I113: CLR   ;
      =     L     20.1;
I114: L     L#8;
      *D    ;
      SPO   I115;
      SPA   I116;
I115: CLR   ;
      =     L     20.1;
I116: LAR1  ;
      L     LB [AR1,P#2.0];
      LAR1  LD    22;
      T     DIB [AR1,P#118.0];
      L     #i;
      L     1;
      +I    ;
      SPO   I117;
      SPA   I118;
I117: CLR   ;
      =     L     20.1;
I118: T     #i;
      SPA   A7fe;
A7ff: L     #PAR_CHANGE_IN.PARVAL;
      T     #TMP_VAL;
      L     0;
      T     #i;
A800: L     #i;
      L     3;
      <=I   ;
      SPBN  A801;
      L     26;
      L     #i;
      +I    ;
      SPO   I119;
      SPA   I11a;
I119: CLR   ;
      =     L     20.1;
I11a: ITD   ;
      L     L#0;
      >=D   ;
      U     L     20.1;
      =     L     20.1;
      TAK   ;
      L     L#31;
      <=D   ;
      U     L     20.1;
      =     L     20.1;
      TAK   ;
      L     L#8;
      *D    ;
      SPO   I11b;
      SPA   I11c;
I11b: CLR   ;
      =     L     20.1;
I11c: TAR2  ;
      +D    ;
      SPO   I11d;
      SPA   I11e;
I11d: CLR   ;
      =     L     20.1;
I11e: L     1;
      TAK   ;
      T     LD    22;
      TAK   ;
      L     #i;
      +I    ;
      SPO   I11f;
      SPA   I120;
I11f: CLR   ;
      =     L     20.1;
I120: ITD   ;
      L     L#1;
      >=D   ;
      U     L     20.1;
      =     L     20.1;
      TAK   ;
      L     L#4;
      <=D   ;
      U     L     20.1;
      =     L     20.1;
      TAK   ;
      L     L#1;
      -D    ;
      SPO   I121;
      SPA   I122;
I121: CLR   ;
      =     L     20.1;
I122: L     L#8;
      *D    ;
      SPO   I123;
      SPA   I124;
I123: CLR   ;
      =     L     20.1;
I124: LAR1  ;
      L     LB [AR1,P#2.0];
      LAR1  LD    22;
      T     DIB [AR1,P#118.0];
      L     #i;
      L     1;
      +I    ;
      SPO   I125;
      SPA   I126;
I125: CLR   ;
      =     L     20.1;
I126: T     #i;
      SPA   A800;
A801: L     #ADR_OUT;
      T     #ADRE;
      CLR   ;
      U     L     20.1;
      SAVE  ;

      CALL SFC   15 (
           LADDR                    := #ADRE,
           RECORD                   := #DATA_OUT,
           RET_VAL                  := #RET_VAL_TMP);

      L     #RET_VAL_TMP;
      L     0;
      <>I   ;
      =     #SND_ERROR;
      U     #DERROR;
      =     L      8.0;
      U     #CHKERROR;
      =     L      8.1;
      U     #BUFFERR0V;
      =     L      8.2;
      U     #RCV_ERROR;
      =     L      8.3;
      U     #SND_ERROR;
      =     L      8.4;
      U     #LIVEBIT_ERROR;
      =     L      8.5;
      CLR   ;
      =     L      8.6;
      =     L      8.7;
      L     #TMP_BYTE;
      T     #BUS_ERROR_CODE;
      L     B#16#0;
      ==I   ;
      =     #BUS_VALID;
      =     #PAR_CHANGE_OUT.BUS_VALID;
      U     L     20.1;
      SAVE  ;
      BE    ;
END_FUNCTION_BLOCK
